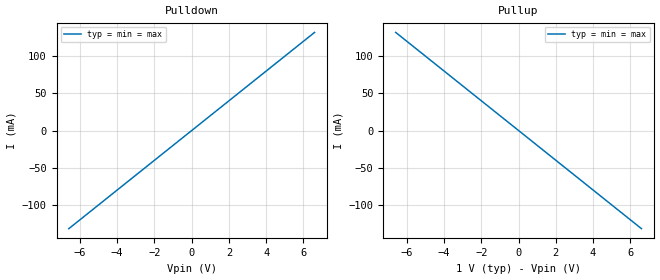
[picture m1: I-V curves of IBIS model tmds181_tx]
[IBIS Ver]   5.0
[File Name]   tmds181.ibs
[File Rev]   1.0
[Component]   tmds181
[Manufacturer] My Company
[Package]
R_pkg  0.0   NA   NA
L_pkg  0.0   NA   NA
C_pkg  0.0   NA   NA
[Pin]   signal_name   model_name   R_pin L_pin  C_pin
1p   tmds181_tx_p   tmds181_tx
1n   tmds181_tx_n   tmds181_tx
2p   tmds181_rx_2p   tmds181_rx
2n   tmds181_rx_2n   tmds181_rx
[Diff_Pin] inv_pin vdiff tdelay_typ tdelay_min tdelay_max
1p   1n   NA   NA   NA   NA
2p   2n   NA   NA   NA   NA
[Model] tmds181_rx
Model_type Input
C_comp 0p 0p 0p
Vinh = 0.25
Vinl = -0.25
[Temperature_Range] 25 125 0
[Voltage Range] 1.0 1.0 1.0
[Algorithmic Model]
Executable Windows_cl16.00.30319.01_64 tmds181_rx_x64.dll tmds181_rx.ami
Executable Windows_cl16.00.30319.01_32 tmds181_rx.dll tmds181_rx.ami
[End Algorithmic Model]
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| Models and submodels in the file (2): tmds181_tx (Output), tmds181_rx (Input)
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[Model] tmds181_tx
Model_type Output
C_comp 0p 0p 0p
Cref = 0
Vref = 0.5
Rref = 50
Vmeas = 0.5
[Temperature_Range] 25 125 0
[Voltage Range] 1.0 1.0 1.0
[Algorithmic Model]
Executable Windows_cl16.00.30319.01_64 tmds181_tx_x64.dll tmds181_tx.ami
Executable Windows_cl16.00.30319.01_32 tmds181_tx.dll tmds181_tx.ami
[End Algorithmic Model]
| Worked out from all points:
|   slope of the pulldown table from 0 to 0.15 V, typ, clamps not added: 50 ohm
|   slope of the pullup table from 0 to 0.15 V, typ, clamps not added: 50 ohm
[Pulldown]
-6.6V     -132mA     -132mA     -132mA
0V        0A         0A         0A
6.6V      132mA      132mA      132mA
[Pullup]
-6.6V     132mA      132mA      132mA
0V        0A         0A         0A
6.6V      -132mA     -132mA     -132mA
[GND Clamp]
-6.6V     0A         0A         0A
0V        0A         0A         0A
6.6V      0A         0A         0A
[Power Clamp]
-6.6V     0A         0A         0A
0V        0A         0A         0A
6.6V      0A         0A         0A
[Ramp]
dV/dt_r 0.3/1.5p 0.3/1.5p 0.3/1.5p
dV/dt_f 0.3/1.5p 0.3/1.5p 0.3/1.5p
